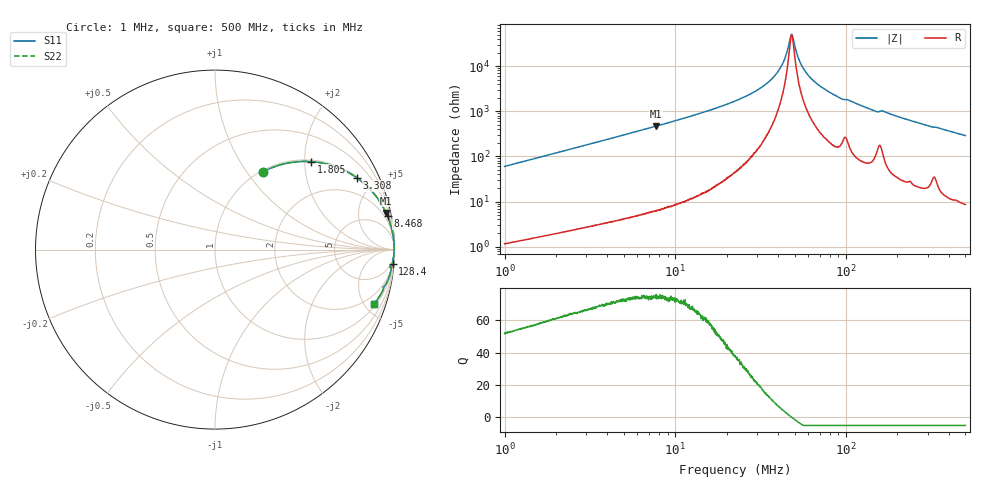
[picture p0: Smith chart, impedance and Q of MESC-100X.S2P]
!s-Parameter Generated by FASTRON Sdn. Bhd.
!FASTRON P/N : MESC-100X
!Keysight Technologies,E4991B,MY54100416,A.01.15
!Date: Mon Mar 16 10:53:48 2026
!Version  : Rev00 Mon Mar 16 10:53:48 2026
!Data & Calibration Information:
!PortZ  Port1:50+j0  Port2:50+j0
!When reading, reference impedance value at option line is always used.
! Remarks : This data is being provided solely for informational purposes.
!Freq	S11	S21	S12	S22
# Hz S dB R 50
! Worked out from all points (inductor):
!   1601 points, 1 MHz to 500 MHz, reference 50 ohm
!   read as one part in series: L = 9.51 uH near 1.032 MHz
!   highest Q = 75.1 at 7.714 MHz (marker M1), where L = 9.62 uH
!   self-resonance near 47.88 MHz
!   S11 on the Smith chart (normalised r, x): 1 MHz: 1.02, +1.20; 1.805 MHz: 1.04, +2.15; 3.308 MHz: 1.06, +3.94; 8.468 MHz: 1, +10; 128.4 MHz: 2, -25; 500 MHz: 1.17, -5.78
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1000000  -5.85 58.2  -1.41 -30.6  -1.41 -30.6  -5.85 58.2
1804688  -2.78 42.5  -3.41 -46.6  -3.41 -46.6  -2.78 42.5
2820919  -1.38 30.6  -5.87 -58.6  -5.87 -58.6  -1.38 30.6
3307895  -1.05 26.8  -6.93 -62.4  -6.93 -62.4  -1.05 26.8
7714120  -0.22 12.1  -13.60 -77.2  -13.60 -77.2  -0.22 12.1
7957584  -0.21 11.7  -13.87 -77.5  -13.87 -77.5  -0.21 11.7
8467807  -0.18 11.0  -14.41 -78.3  -14.41 -78.3  -0.18 11.0
2.236068e7  -0.03 3.4  -24.53 -85.1  -24.53 -85.1  -0.03 3.4
3.050939e7  -0.02 1.9  -29.58 -85.3  -29.58 -85.3  -0.02 1.9
3.777553e7  -0.02 1.0  -35.29 -83.1  -35.29 -83.1  -0.02 1.0
4.2775e7  -0.02 0.5  -41.51 -76.7  -41.51 -76.7  -0.02 0.5
4.464218e7  -0.02 0.3  -45.19 -69.3  -45.19 -69.3  -0.02 0.3
4.695421e7  -0.02 0.1  -51.81 -38.6  -51.81 -38.6  -0.02 0.1
4.7875e7  -0.02 0.0  -53.89 -6.2  -53.89 -6.2  -0.02 0.0
4.900382e7  -0.02 -0.1  -52.20 34.2  -52.20 34.2  -0.02 -0.1
5.194369e7  -0.02 -0.3  -44.65 69.2  -44.65 69.2  -0.02 -0.3
5.442207e7  -0.02 -0.5  -40.91 75.6  -40.91 75.6  -0.02 -0.5
6.307767e7  -0.02 -1.1  -34.19 81.7  -34.19 81.7  -0.02 -1.1
9.122775e7  -0.05 -2.8  -26.08 82.4  -26.08 82.4  -0.05 -2.8
1.284016e8  -0.07 -4.6  -21.98 82.1  -21.98 82.1  -0.07 -4.6
1.77937e8  -0.11 -6.3  -19.13 80.4  -19.13 80.4  -0.11 -6.3
5e8  -0.57 -18.9  -9.79 69.4  -9.79 69.4  -0.57 -18.9
